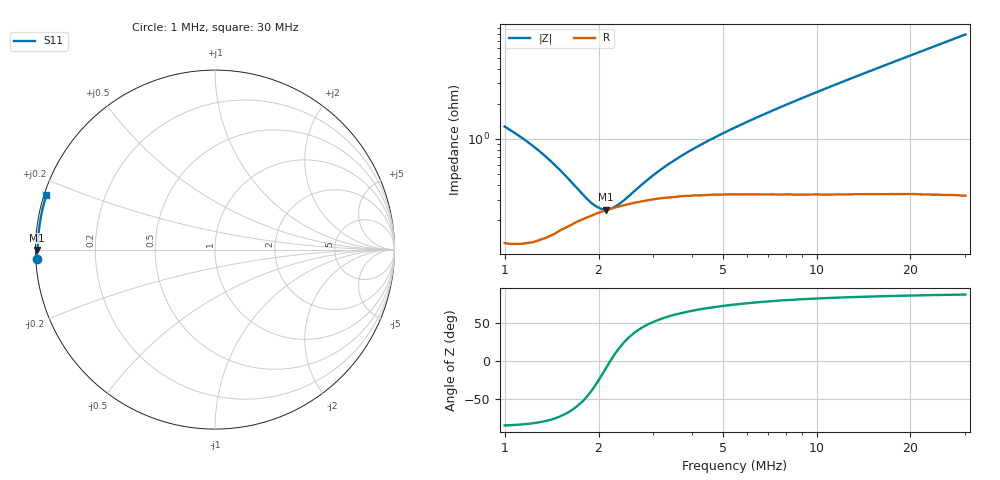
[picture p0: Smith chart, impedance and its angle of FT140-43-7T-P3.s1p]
! ListType=Log
!!FT140-43 7T Port 3
# MHz S DB R 50
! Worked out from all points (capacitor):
!   101 points, 1 MHz to 30 MHz, reference 50 ohm
!   read as one part to ground: C = 99.2 nF near 1 MHz
!   lowest |Z| = 247 mohm at 2.113 MHz (marker M1)
!   series resonance near 2.179 MHz, so ESL is about 54 nH
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1  -0.04 -177.1
1.107423  -0.04 -177.6
1.226386  -0.04 -178.0
1.312713  -0.05 -178.3
1.453729  -0.05 -178.7
1.556058  -0.06 -178.9
1.723215  -0.07 -179.3
1.908328  -0.08 -179.6
2.113327  -0.08 -179.9
2.340347  -0.09 -180.2
2.591755  -0.10 -180.5
2.87017  -0.10 -180.8
3.178493  -0.11 -181.0
3.89806  -0.11 -181.6
4.780527  -0.12 -182.3
6.275459  -0.12 -183.3
8.52288  -0.12 -184.8
10.45234  -0.12 -186.0
11.97563  -0.12 -187.0
13.72092  -0.12 -188.0
15.72057  -0.12 -189.3
16.82715  -0.12 -190.0
19.27949  -0.12 -191.5
21.35055  -0.11 -192.7
22.85344  -0.11 -193.6
25.30843  -0.11 -195.1
27.08991  -0.11 -196.2
30  -0.11 -198.0
